ORGANIZATION_BLOCK "COMPLETE RESTART"
TITLE = "Complete Restart"
VERSION : 0.1


VAR_TEMP
  OB100_EV_CLASS : BYTE ;	//16#13, Event class 1, Entering event state, Event logged in diagnostic buffer
  OB100_STRTUP : BYTE ;	//16#81/82/83/84 Method of startup
  OB100_PRIORITY : BYTE ;	//27 (Priority of 1 is lowest)
  OB100_OB_NUMBR : BYTE ;	//100 (Organization block 100, OB100)
  OB100_RESERVED_1 : BYTE ;	//Reserved for system
  OB100_RESERVED_2 : BYTE ;	//Reserved for system
  OB100_STOP : WORD ;	//Event that caused CPU to stop (16#4xxx)
  OB100_STRT_INFO : DWORD ;	//Information on how system started
  OB100_DATE_TIME : DATE_AND_TIME ;	//Date and time OB100 started
END_VAR
BEGIN
NETWORK
TITLE =

      U     "START CICLO ASPO";
      O     "START CICLO PROFILA";
      R     "START CICLO ASPO";
      R     "START CICLO PROFILA";

END_ORGANIZATION_BLOCK

